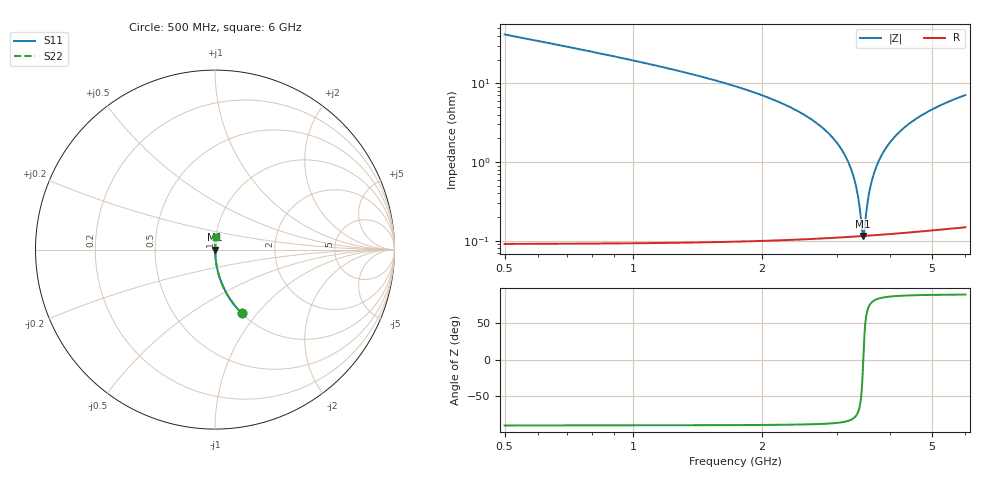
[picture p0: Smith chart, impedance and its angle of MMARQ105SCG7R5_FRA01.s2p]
! MMARQ105SCG7R5_FRA01  S-PARAMETER MODEL  ( General Type )
! Model Generated by TAIYO YUDEN Corporation (http://www.ty-top.com)
! Version 1.0
! TAIYO YUDEN Control No. 200326
! Copyright(c) 2020 TAIYO YUDEN CO.,LTD. All Rights Reserved.
! Product Description (link to TY-COMPAS)
! https://ds.yuden.co.jp/TYCOMPAS/or/detail?pn=MMARQ105SCG7R5CFRA01&u=M
! Products Name : Multilayer Ceramic Capacitors
! Characteristics :
!  Capacitance : 7.5 pF , Rated Voltage : 250V , TCC : CG / C0G
!  Case Size : 1.0 x 0.5 / 0.039 x 0.02 [mm/inch] , Thickness : 0.5 / 0.02 [mm/inch]
!  (Conditions: Temperature = 25 degC , DC Bias Current/Voltage = 0A / 0V)
! External Node Assignments :
!  1  o---| |---o  2
! GND o---------o GND
! Frequency Range : 500MHz  -  6GHz  [ 401 STEP ]
# MHz S RI R 50
! Freq[MHz].  S11 Real  S11 Imag  S21 Real  S21 Imag  S12 Real  S12 Imag  S22 Real  S22 Imag
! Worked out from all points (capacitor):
!   401 points, 500 MHz to 6 GHz, reference 50 ohm
!   read as one part in series: C = 7.49 pF near 527.5 MHz
!   lowest |Z| = 116 mohm at 3.456 GHz (marker M1)
!   series resonance near 3.459 GHz, so ESL is about 280 pH
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500  0.1482 -0.3542  0.8518 0.3542  0.8518 0.3542  0.1482 -0.3542
830  0.0558 -0.2277  0.9442 0.2277  0.9442 0.2277  0.0558 -0.2277
1421.25  0.0161 -0.1222  0.9839 0.1222  0.9839 0.1222  0.0161 -0.1222
2342.5  0.00342 -0.0489  0.9966 0.0489  0.9966 0.0489  0.00342 -0.0489
2672.5  0.00208 -0.0319  0.9979 0.0319  0.9979 0.0319  0.00208 -0.0319
2920  0.00152 -0.0209  0.9985 0.0209  0.9985 0.0209  0.00152 -0.0209
3112.5  0.00128 -0.013  0.9987 0.013  0.9987 0.013  0.00128 -0.013
3250  0.00118 -0.00765  0.9988 0.00765  0.9988 0.00765  0.00118 -0.00765
3346.25  0.00115 -0.00407  0.9988 0.00407  0.9988 0.00407  0.00115 -0.00407
3387.5  0.00115 -0.00257  0.9989 0.00257  0.9989 0.00257  0.00115 -0.00257
3428.75  0.00115 -0.00109  0.9989 0.00109  0.9989 0.00109  0.00115 -0.00109
3456.25  0.00115 -0.000107  0.9989 0.000107  0.9989 0.000107  0.00115 -0.000107
3483.75  0.00115 0.000863  0.9988 -0.000863  0.9988 -0.000863  0.00115 0.000863
3538.75  0.00117 0.00278  0.9988 -0.00278  0.9988 -0.00278  0.00117 0.00278
3580  0.00118 0.0042  0.9988 -0.0042  0.9988 -0.0042  0.00118 0.0042
3635  0.00121 0.00607  0.9988 -0.00607  0.9988 -0.00607  0.00121 0.00607
3703.75  0.00125 0.00837  0.9987 -0.00837  0.9987 -0.00837  0.00125 0.00837
3896.25  0.00142 0.0146  0.9986 -0.0146  0.9986 -0.0146  0.00142 0.0146
4171.25  0.00177 0.023  0.9982 -0.023  0.9982 -0.023  0.00177 0.023
4570  0.00248 0.0345  0.9975 -0.0345  0.9975 -0.0345  0.00248 0.0345
5092.5  0.00371 0.0484  0.9963 -0.0484  0.9963 -0.0484  0.00371 0.0484
6000  0.00647 0.0704  0.9935 -0.0704  0.9935 -0.0704  0.00647 0.0704
